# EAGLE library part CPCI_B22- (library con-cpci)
Compact PCI B 22 Source: www.erni.com
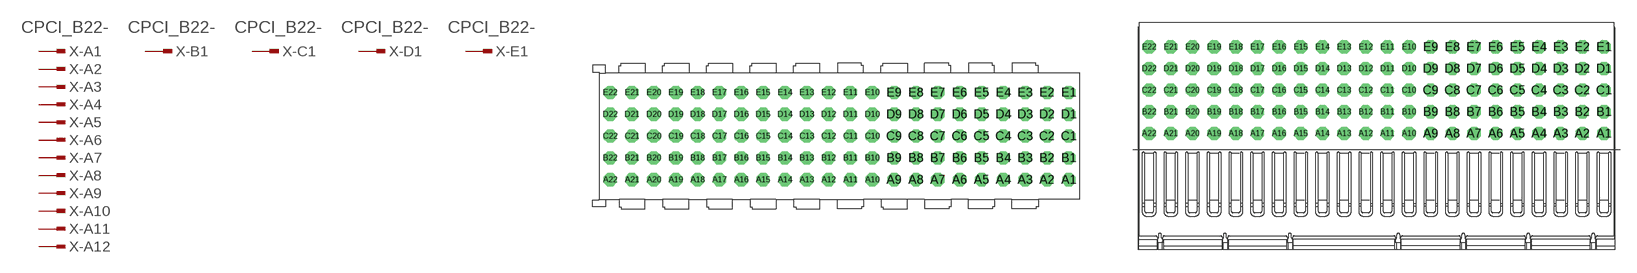
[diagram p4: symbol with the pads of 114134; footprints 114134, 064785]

Designator prefix X; gates -A1=PINV -B1=PINV -C1=PINV -D1=PINV -E1=PINV -A2=PIN -A3=PIN -A4=PIN -A5=PIN -A6=PIN -A7=PIN -A8=PIN -A9=PIN -A10=PIN -A11=PIN -A12=PIN -A13=PIN -A14=PIN -A15=PIN -A16=PIN -A17=PIN -A18=PIN -A19=PIN -A20=PIN -A21=PIN -A22=PIN -B2=PIN -B3=PIN -B4=PIN -B5=PIN -B6=PIN -B7=PIN -B8=PIN -B9=PIN -B10=PIN -B11=PIN -B12=PIN -B13=PIN -B14=PIN -B15=PIN -B16=PIN -B17=PIN -B18=PIN -B19=PIN -B20=PIN -B21=PIN -B22=PIN -C2=PIN -C3=PIN -C4=PIN -C5=PIN -C6=PIN -C7=PIN -C8=PIN -C9=PIN -C10=PIN -C11=PIN -C12=PIN -C13=PIN -C14=PIN -C15=PIN -C16=PIN -C17=PIN -C18=PIN -C19=PIN -C20=PIN -C21=PIN -C22=PIN -D2=PIN -D3=PIN -D4=PIN -D5=PIN -D6=PIN -D7=PIN -D8=PIN -D9=PIN -D10=PIN -D11=PIN -D12=PIN -D13=PIN -D14=PIN -D15=PIN -D16=PIN -D17=PIN -D18=PIN -D19=PIN -D20=PIN -D21=PIN -D22=PIN -E2=PIN -E3=PIN -E4=PIN -E5=PIN -E6=PIN -E7=PIN -E8=PIN -E9=PIN -E10=PIN -E11=PIN -E12=PIN -E13=PIN -E14=PIN -E15=PIN -E16=PIN -E17=PIN -E18=PIN -E19=PIN -E20=PIN -E21=PIN -E22=PIN

## CPCI_B22-114134 (OC_FARNELL: unknown; OC_NEWARK: unknown)  [114134]
A1  -A1:1  in
A2  -A2:1  in
A3  -A3:1  in
A4  -A4:1  in
A5  -A5:1  in
A6  -A6:1  in
A7  -A7:1  in
A8  -A8:1  in
A9  -A9:1  in
A10  -A10:1  in
A11  -A11:1  in
A12  -A12:1  in
A13  -A13:1  in
A14  -A14:1  in
A15  -A15:1  in
A16  -A16:1  in
A17  -A17:1  in
A18  -A18:1  in
A19  -A19:1  in
A20  -A20:1  in
A21  -A21:1  in
A22  -A22:1  in
B1  -B1:1  in
B2  -B2:1  in
B3  -B3:1  in
B4  -B4:1  in
B5  -B5:1  in
B6  -B6:1  in
B7  -B7:1  in
B8  -B8:1  in
B9  -B9:1  in
B10  -B10:1  in
B11  -B11:1  in
B12  -B12:1  in
B13  -B13:1  in
B14  -B14:1  in
B15  -B15:1  in
B16  -B16:1  in
B17  -B17:1  in
B18  -B18:1  in
B19  -B19:1  in
B20  -B20:1  in
B21  -B21:1  in
B22  -B22:1  in
C1  -C1:1  in
C2  -C2:1  in
C3  -C3:1  in
C4  -C4:1  in
C5  -C5:1  in
C6  -C6:1  in
C7  -C7:1  in
C8  -C8:1  in
C9  -C9:1  in
C10  -C10:1  in
C11  -C11:1  in
C12  -C12:1  in
C13  -C13:1  in
C14  -C14:1  in
C15  -C15:1  in
C16  -C16:1  in
C17  -C17:1  in
C18  -C18:1  in
C19  -C19:1  in
C20  -C20:1  in
C21  -C21:1  in
C22  -C22:1  in
D1  -D1:1  in
D2  -D2:1  in
D3  -D3:1  in
D4  -D4:1  in
D5  -D5:1  in
D6  -D6:1  in
D7  -D7:1  in
D8  -D8:1  in
D9  -D9:1  in
D10  -D10:1  in
D11  -D11:1  in
D12  -D12:1  in
D13  -D13:1  in
D14  -D14:1  in
D15  -D15:1  in
D16  -D16:1  in
D17  -D17:1  in
D18  -D18:1  in
D19  -D19:1  in
D20  -D20:1  in
D21  -D21:1  in
D22  -D22:1  in
E1  -E1:1  in
E2  -E2:1  in
E3  -E3:1  in
E4  -E4:1  in
E5  -E5:1  in
E6  -E6:1  in
E7  -E7:1  in
E8  -E8:1  in
E9  -E9:1  in
E10  -E10:1  in
E11  -E11:1  in
E12  -E12:1  in
E13  -E13:1  in
E14  -E14:1  in
E15  -E15:1  in
E16  -E16:1  in
E17  -E17:1  in
E18  -E18:1  in
E19  -E19:1  in
E20  -E20:1  in
E21  -E21:1  in
E22  -E22:1  in

## CPCI_B22-064785 (OC_FARNELL: unknown; OC_NEWARK: unknown)  [064785]
Pads as for 114134

## CPCI_B22-914797I (OC_FARNELL: unknown; OC_NEWARK: unknown)  [914797I]
Pads as for 114134

## Footprint 114134 (pad centres in mm)
ERmet-FS Federleiste B22 / ERmet-Female Straight Type B22 Source: http://www.erni.com/DB/PDF-Drawing/ERmet/114134.pdf
drill 0.7 pad 1.016 octagon: A1 21,-4; A2 19,-4; A3 17,-4; A4 15,-4; A5 13,-4; A6 11,-4; A7 9,-4; A8 7,-4; A9 5,-4; A10 3,-4; A11 1,-4; A12 -1,-4; A13 -3,-4; A14 -5,-4; A15 -7,-4; A16 -9,-4; A17 -11,-4; A18 -13,-4; A19 -15,-4; A20 -17,-4; A21 -19,-4; A22 -21,-4; B1 21,-2; B2 19,-2; B3 17,-2; B4 15,-2; B5 13,-2; B6 11,-2; B7 9,-2; B8 7,-2; B9 5,-2; B10 3,-2; B11 1,-2; B12 -1,-2; B13 -3,-2; B14 -5,-2; B15 -7,-2; B16 -9,-2; B17 -11,-2; B18 -13,-2; B19 -15,-2; B20 -17,-2; B21 -19,-2; B22 -21,-2; C1 21,0; C2 19,0; C3 17,0; C4 15,0; C5 13,0; C6 11,0; C7 9,0; C8 7,0; C9 5,0; C10 3,0; C11 1,0; C12 -1,0; C13 -3,0; C14 -5,0; C15 -7,0; C16 -9,0; C17 -11,0; C18 -13,0; C19 -15,0; C20 -17,0; C21 -19,0; C22 -21,0; D1 21,2; D2 19,2; D3 17,2; D4 15,2; D5 13,2; D6 11,2; D7 9,2; D8 7,2; D9 5,2; D10 3,2; D11 1,2; D12 -1,2; D13 -3,2; D14 -5,2; D15 -7,2; D16 -9,2; D17 -11,2; D18 -13,2; D19 -15,2; D20 -17,2; D21 -19,2; D22 -21,2; E1 21,4; E2 19,4; E3 17,4; E4 15,4; E5 13,4; E6 11,4; E7 9,4; E8 7,4; E9 5,4; E10 3,4; E11 1,4; E12 -1,4; E13 -3,4; E14 -5,4; E15 -7,4; E16 -9,4; E17 -11,4; E18 -13,4; E19 -15,4; E20 -17,4; E21 -19,4; E22 -21,4

## Footprint 064785 (pad centres in mm)
ERmet Federleiste B 22 / ERmet Female Type B 22 Source: http://www.erni.com/DB/PDF-Drawing/ERmet/064785.pdf
drill 0.7 pad 1.016 octagon: A1 21,0; A2 19,0; A3 17,0; A4 15,0; A5 13,0; A6 11,0; A7 9,0; A8 7,0; A9 5,0; A10 3,0; A11 1,0; A12 -1,0; A13 -3,0; A14 -5,0; A15 -7,0; A16 -9,0; A17 -11,0; A18 -13,0; A19 -15,0; A20 -17,0; A21 -19,0; A22 -21,0; B1 21,2; B2 19,2; B3 17,2; B4 15,2; B5 13,2; B6 11,2; B7 9,2; B8 7,2; B9 5,2; B10 3,2; B11 1,2; B12 -1,2; B13 -3,2; B14 -5,2; B15 -7,2; B16 -9,2; B17 -11,2; B18 -13,2; B19 -15,2; B20 -17,2; B21 -19,2; B22 -21,2; C1 21,4; C2 19,4; C3 17,4; C4 15,4; C5 13,4; C6 11,4; C7 9,4; C8 7,4; C9 5,4; C10 3,4; C11 1,4; C12 -1,4; C13 -3,4; C14 -5,4; C15 -7,4; C16 -9,4; C17 -11,4; C18 -13,4; C19 -15,4; C20 -17,4; C21 -19,4; C22 -21,4; D1 21,6; D2 19,6; D3 17,6; D4 15,6; D5 13,6; D6 11,6; D7 9,6; D8 7,6; D9 5,6; D10 3,6; D11 1,6; D12 -1,6; D13 -3,6; D14 -5,6; D15 -7,6; D16 -9,6; D17 -11,6; D18 -13,6; D19 -15,6; D20 -17,6; D21 -19,6; D22 -21,6; E1 21,8; E2 19,8; E3 17,8; E4 15,8; E5 13,8; E6 11,8; E7 9,8; E8 7,8; E9 5,8; E10 3,8; E11 1,8; E12 -1,8; E13 -3,8; E14 -5,8; E15 -7,8; E16 -9,8; E17 -11,8; E18 -13,8; E19 -15,8; E20 -17,8; E21 -19,8; E22 -21,8

## Footprint 914797I (pad centres in mm)
ERmet Federleiste B 22 / ERmet Female Type B 22 Source: http://www.erni.com/DB/PDF-Drawing/ERmet/914797.pdf
drill 0.7 pad 1.016 octagon: A1 21,0; A2 19,0; A3 17,0; A4 15,0; A5 13,0; A6 11,0; A7 9,0; A8 7,0; A9 5,0; A10 3,0; A11 1,0; A12 -1,0; A13 -3,0; A14 -5,0; A15 -7,0; A16 -9,0; A17 -11,0; A18 -13,0; A19 -15,0; A20 -17,0; A21 -19,0; A22 -21,0; B1 21,2; B2 19,2; B3 17,2; B4 15,2; B5 13,2; B6 11,2; B7 9,2; B8 7,2; B9 5,2; B10 3,2; B11 1,2; B12 -1,2; B13 -3,2; B14 -5,2; B15 -7,2; B16 -9,2; B17 -11,2; B18 -13,2; B19 -15,2; B20 -17,2; B21 -19,2; B22 -21,2; C1 21,4; C2 19,4; C3 17,4; C4 15,4; C5 13,4; C6 11,4; C7 9,4; C8 7,4; C9 5,4; C10 3,4; C11 1,4; C12 -1,4; C13 -3,4; C14 -5,4; C15 -7,4; C16 -9,4; C17 -11,4; C18 -13,4; C19 -15,4; C20 -17,4; C21 -19,4; C22 -21,4; D1 21,6; D2 19,6; D3 17,6; D4 15,6; D5 13,6; D6 11,6; D7 9,6; D8 7,6; D9 5,6; D10 3,6; D11 1,6; D12 -1,6; D13 -3,6; D14 -5,6; D15 -7,6; D16 -9,6; D17 -11,6; D18 -13,6; D19 -15,6; D20 -17,6; D21 -19,6; D22 -21,6; E1 21,8; E2 19,8; E3 17,8; E4 15,8; E5 13,8; E6 11,8; E7 9,8; E8 7,8; E9 5,8; E10 3,8; E11 1,8; E12 -1,8; E13 -3,8; E14 -5,8; E15 -7,8; E16 -9,8; E17 -11,8; E18 -13,8; E19 -15,8; E20 -17,8; E21 -19,8; E22 -21,8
